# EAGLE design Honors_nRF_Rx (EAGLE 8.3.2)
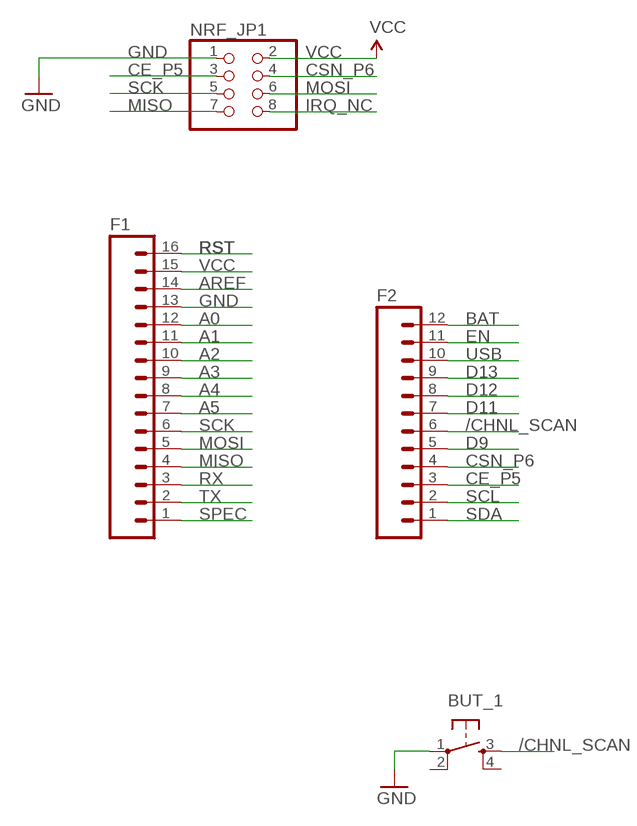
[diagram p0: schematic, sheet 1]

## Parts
BUT_1  TAC_SWITCHPTH  [TACTILE-PTH]
F1  M16PTH  [1X16]
F2  M12PTH  [1X12]
NRF_JP1  PINHD-2X4  [2X04]

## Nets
/CHNL_SCAN: BUT_1.3 F2.6
A0: F1.12
A1: F1.11
A2: F1.10
A3: F1.9
A4: F1.8
A5: F1.7
AREF: F1.14
BAT: F2.12
CE_P5: F2.3 NRF_JP1.3
CSN_P6: F2.4 NRF_JP1.4
D9: F2.5
D11: F2.7
D12: F2.8
D13: F2.9
EN: F2.11
GND: BUT_1.1 F1.13 NRF_JP1.1
IRQ_NC: NRF_JP1.8
MISO: F1.4 NRF_JP1.7
MOSI: F1.5 NRF_JP1.6
RST: F1.16
RX: F1.3
SCK: F1.6 NRF_JP1.5
SCL: F2.2
SDA: F2.1
SPEC: F1.1
TX: F1.2
USB: F2.10
VCC: F1.15 NRF_JP1.2
Unconnected: BUT_1.2 BUT_1.4

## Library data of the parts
BUT_1 = SparkFun-Retired:TAC_SWITCH: Momentary Switch Button commonly used for reset or general input. Spark Fun Electronics SKU : COM-00097 SMT- SWCH-08247
F1 = SparkFun-Connectors:M16: 1x16 .1" header
F2 = SparkFun-Connectors:M12: Header 12 Standard 12-pin 0.1" header. Use with straight break away headers (SKU : PRT-00116), right angle break away headers (PRT-00553), swiss pins (PRT-00743), machine pins (PRT-00117), and female headers (PRT-00115).
NRF_JP1 = pinhead:PINHD-2X4: PIN HEADER

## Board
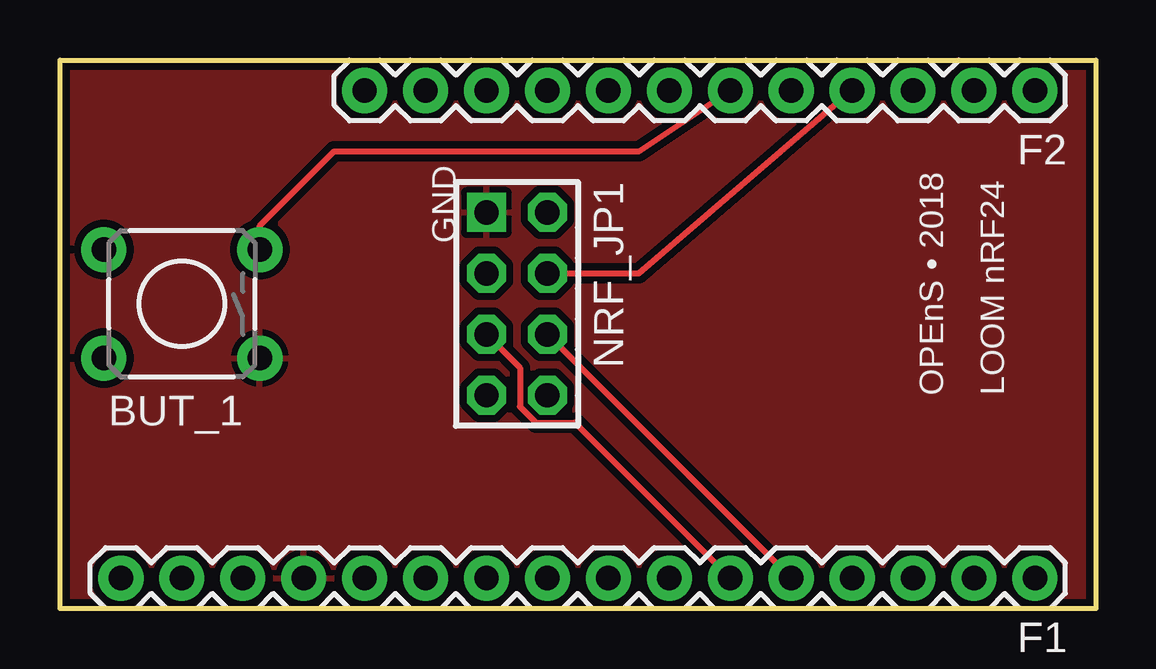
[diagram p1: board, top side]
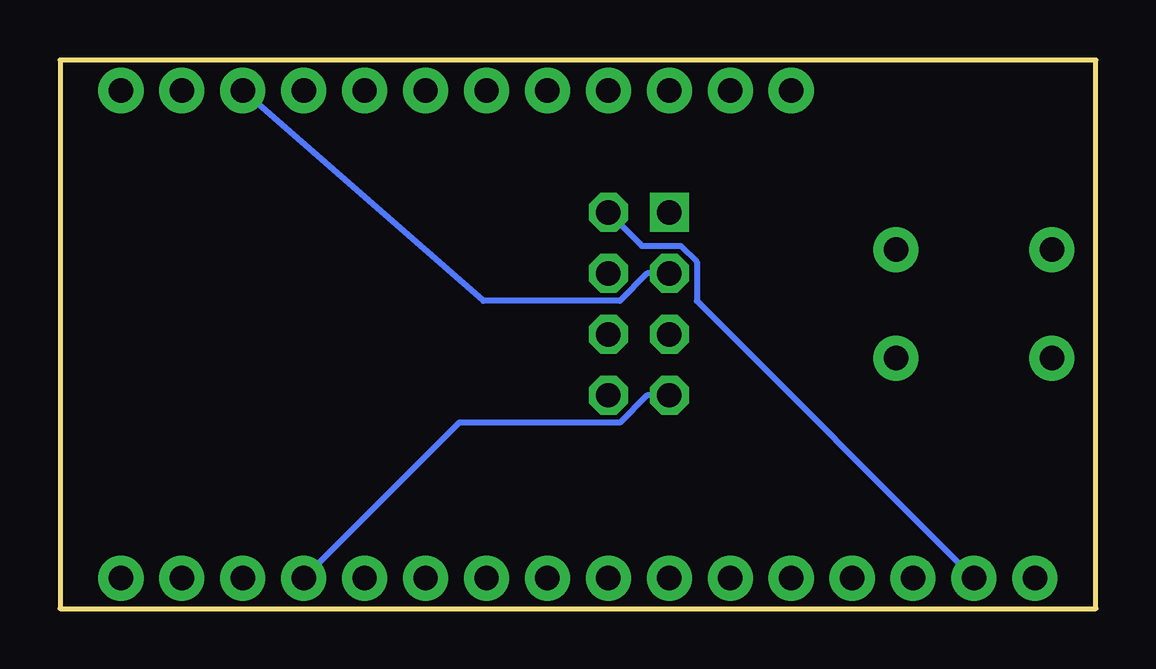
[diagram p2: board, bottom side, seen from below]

Size 43.18 x 22.86 mm. Coordinates in mm from the lower left corner, seen from the top.
Outline: 0,0 0,22.86 43.18,22.86 43.18,0 0,0
Copper layers (1*16): Top 0.035mm / dielectric 1.5mm / Bottom 0.035mm
Design rules "SparkFun": minimum track width 8mil, minimum drill 20mil, track to track 8mil, track to pad 8mil, pad to pad 8mil, via to via 8mil, smd to smd 8mil, copper to edge 8mil, drill to drill 8mil, minimum pad ring 12mil, minimum via ring 10mil, stop-mask expansion 4mil, vias tented up to drill 20mil, thermal gap 10mil

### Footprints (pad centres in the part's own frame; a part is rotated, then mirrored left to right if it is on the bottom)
TACTILE-PTH = drill 1.016 pad 1.88: 1 -3.251,2.261; 2 3.251,2.261; 3 -3.251,-2.261; 4 3.251,-2.261
1X16 = drill 1.016 pad 1.88: 1 0,0; 2 2.54,0; 3 5.08,0; 4 7.62,0; 5 10.16,0; 6 12.7,0; 7 15.24,0; 8 17.78,0; 9 20.32,0; 10 22.86,0; 11 25.4,0; 12 27.94,0; 13 30.48,0; 14 33.02,0; 15 35.56,0; 16 38.1,0
1X12 = drill 1.016 pad 1.88: 1 0,0; 2 2.54,0; 3 5.08,0; 4 7.62,0; 5 10.16,0; 6 12.7,0; 7 15.24,0; 8 17.78,0; 9 20.32,0; 10 22.86,0; 11 25.4,0; 12 27.94,0
2X04 = drill 1.016 square: 1 -3.81,-1.27 | drill 1.016 octagon: 2 -3.81,1.27; 3 -1.27,-1.27; 4 -1.27,1.27; 5 1.27,-1.27; 6 1.27,1.27; 7 3.81,-1.27; 8 3.81,1.27

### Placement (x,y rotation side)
BUT_1  5.08,12.7 180 top
F1  40.64,1.27 180 top
F2  40.64,21.59 180 top
NRF_JP1  19.05,12.7 270 top

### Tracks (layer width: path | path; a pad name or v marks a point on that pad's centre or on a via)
/CHNL_SCAN
  Top 0.254: BUT_1.3 8.33,15.95 11.43,19.05 24.13,19.05 F2.6
CE_P5
  Bottom 0.254: NRF_JP1.3 18.7,13.97 19.85,12.83 25.53,12.83 F2.3
CSN_P6
  Top 0.254: NRF_JP1.4 24.13,13.97 F2.4
GND
  pour Top (isolate 0.305): 0,0 0,22.86 43.18,22.86 43.18,0
MISO
  Bottom 0.254: NRF_JP1.7 18.7,8.89 19.85,7.75 26.54,7.75 F1.4
MOSI
  Top 0.254: NRF_JP1.6 F1.5
SCK
  Top 0.254: NRF_JP1.5 19.18,10.03 19.18,8.42 19.85,7.75 21.46,7.75 F1.6
VCC
  Bottom 0.254: NRF_JP1.2 18.92,15.11 17.31,15.11 16.64,14.44 16.64,12.83 F1.15

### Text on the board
tPlace: GND | OPEnS • 2018 | LOOM nRF24

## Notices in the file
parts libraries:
SparkFun-Connectors: Licensing: Creative Commons ShareAlike 4.0 International - https://creativecommons.org/licenses/by-sa/4.0
